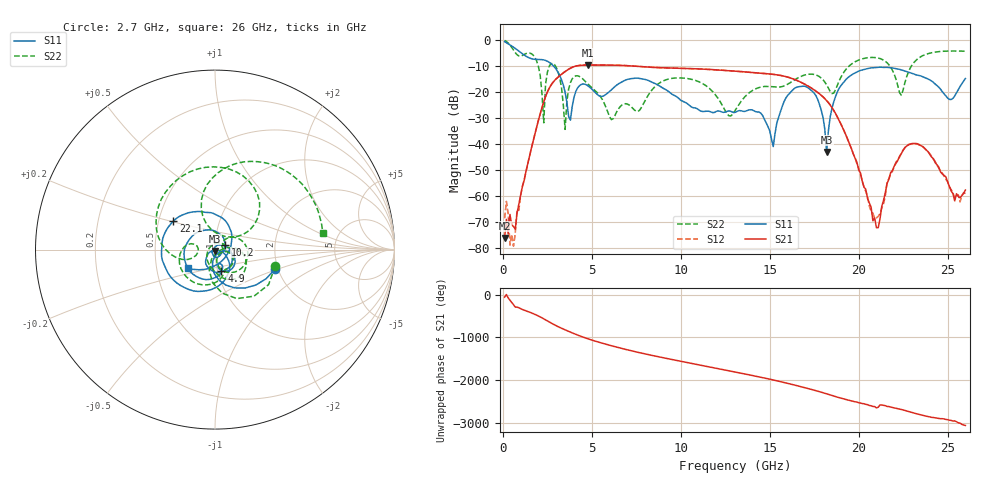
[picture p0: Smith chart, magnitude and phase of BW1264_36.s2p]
!Keysight Technologies,N5245B,MY57181159,A.13.60.06
!Date: Friday, December 18, 2020 23:53:50
!Correction: S11(Full 2 Port(1,2))
!S21(Full 2 Port(1,2))
!S12(Full 2 Port(1,2))
!S22(Full 2 Port(1,2))
!S2P File: Measurements: S11, S21, S12, S22:
# Hz S  dB  R 50
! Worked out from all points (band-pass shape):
!   260 points, 100 MHz to 26 GHz, reference 50 ohm
!   highest |S21| = -9.64 dB at 4.8 GHz (marker M1); lowest = -76.1 dB at 100 MHz (marker M2)
!   |S21| within 3 dB of the highest: 3.402 GHz to 14.24 GHz (10.84 GHz wide, 123 % of centre)
!   lowest |S11| = -43.1 dB at 18.2 GHz (marker M3), VSWR 1.01, Z = 50 - j0.703 ohm
!   |S11| at or under -10 dB: 2.844 GHz to end of sweep
!   |S22| runs from -34.4 to -0.2 dB; largest |S21 - S12| = 0.00065
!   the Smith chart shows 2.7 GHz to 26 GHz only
!   S11 on the Smith chart (normalised r, x): 2.7 GHz: 1.94, -0.47; 4.9 GHz: 1.04, -0.25; 10.2 GHz: 1.12, +0.06; 22.1 GHz: 0.60, +0.21; 26 GHz: 0.73, -0.16
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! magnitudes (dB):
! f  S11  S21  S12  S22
! 100 MHz  -0.7  -76.1  -68.5  -0.2
! 600 MHz  -2.8  -71.7  -79.2  -3.9
! 1.9 GHz  -7.5  -33.5  -33.5  -8.1
! 2.3 GHz  -7.7  -23.8  -23.8  -31.8
! 2.7 GHz  -9.1  -17.4  -17.4  -9.2
! 3.5 GHz  -20.1  -12.1  -12.1  -34.4
! 3.8 GHz  -30.8  -10.9  -10.9  -16.4
! 4.5 GHz  -16.9  -9.7  -9.7  -15.0
! 4.8 GHz  -17.7  -9.6  -9.6  -17.1
! 4.9 GHz  -18.3  -9.6  -9.6  -17.7
! 6.1 GHz  -19.2  -9.7  -9.7  -30.6
! 8.8 GHz  -17.7  -10.7  -10.7  -16.6
! 10.2 GHz  -23.8  -10.9  -10.9  -14.7
! 13.1 GHz  -27.7  -12.0  -12.0  -26.6
! 15.2 GHz  -41.0  -13.2  -13.2  -18.0
! 17.4 GHz  -19.7  -18.7  -18.7  -13.2
! 18.2 GHz  -43.1  -23.3  -23.3  -17.2
! 18.9 GHz  -18.6  -30.9  -30.9  -15.8
! 21 GHz  -10.6  -72.1  -68.4  -6.8
! 21.7 GHz  -10.6  -53.5  -53.4  -9.5
! 22.1 GHz  -11.0  -47.4  -46.9  -15.1
! 26 GHz  -14.8  -57.7  -59.0  -4.3
